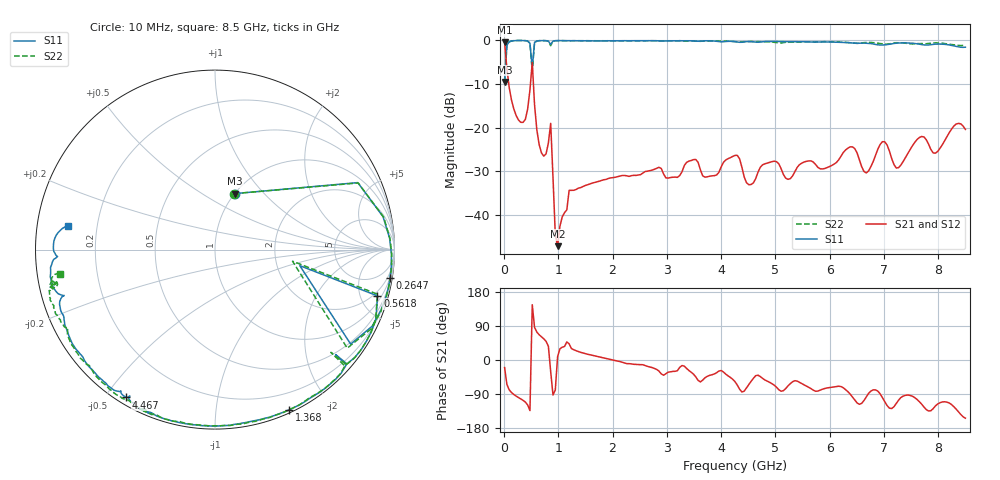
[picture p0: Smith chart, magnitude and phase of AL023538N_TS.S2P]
!AVX CORPORATION
!PN: AL023538N_TS
!DESCRIPTION: AIR CORE INDUCTOR, 538nH, 20 TURNS
!Agilent Technologies,E5071C,MY46102230,A.09.54
!Date: Mon Sep 03 16:52:48 2012
!Data & Calibration Information:
!Freq	S11:SOLT2(ON)	S21:SOLT2(ON)	S12:SOLT2(ON)	S22:SOLT2(ON)
# Hz S dB R 50
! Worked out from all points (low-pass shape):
!   201 points, 10 MHz to 8.5 GHz, reference 50 ohm
!   highest |S21| = -0.48 dB at 10 MHz (marker M1); lowest = -47.1 dB at 986.4 MHz (marker M2)
!   |S21| within 3 dB of the highest: start of sweep to 31.13 MHz
!   lowest |S11| = -9.6 dB at 10 MHz (marker M3), VSWR 1.99, Z = 50.3 + j35.3 ohm
!   |S11| at or under -10 dB: nowhere
!   |S22| runs from -9.6 to -0.1 dB; largest |S21 - S12| = 0.014
!   S11 on the Smith chart (normalised r, x): 10 MHz: 1.01, +0.71; 264.7 MHz: 1, -12; 561.9 MHz: 1.51, -6.84; 1.368 GHz: 0.03, -1.56; 4.467 GHz: 0.03, -0.57; 8.5 GHz: 0.09, +0.08
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1e7  -9.58 70.1  -0.48 -20.1  -0.61 -19.8  -9.63 71.0
5.245e7  -1.12 25.1  -6.51 -64.6  -6.48 -64.7  -1.11 25.0
2.647e8  -0.10 -9.2  -18.23 -98.9  -18.21 -99.1  -0.08 -9.6
4.7695e8  -0.71 -34.9  -11.38 -133.6  -11.37 -133.6  -0.74 -36.7
5.194e8  -6.36 -10.7  -5.09 145.9  -5.09 145.8  -7.19 -8.5
5.6185e8  -0.53 -15.9  -14.81 86.1  -14.80 86.0  -0.55 -15.4
7.3165e8  -0.12 -34.3  -26.50 55.9  -26.52 55.9  -0.12 -34.9
8.59e8  -1.00 -41.0  -19.02 -30.5  -19.02 -30.5  -1.28 -41.6
9.439e8  -0.14 -44.5  -44.41 -79.2  -44.55 -78.7  -0.15 -44.6
9.8635e8  -0.12 -47.0  -47.06 8.8  -47.34 8.4  -0.14 -47.3
1.1986e9  -0.15 -57.6  -34.32 42.7  -34.37 43.0  -0.18 -57.8
1.3684e9  -0.14 -65.1  -33.82 22.3  -33.94 22.2  -0.15 -65.4
1.4533e9  -0.16 -68.7  -33.45 18.7  -33.51 18.8  -0.15 -68.8
2.85415e9  -0.19 -110.3  -29.05 -29.3  -29.06 -29.8  -0.17 -108.3
4.255e9  -0.36 -120.1  -26.34 -57.1  -26.34 -57.3  -0.35 -135.1
4.46725e9  -0.35 -120.9  -32.57 -73.5  -32.60 -73.3  -0.35 -139.2
5.6983e9  -0.46 -140.9  -27.86 -79.6  -27.90 -80.0  -0.44 -160.8
6.41995e9  -0.66 -155.2  -24.39 -97.8  -24.40 -97.7  -0.68 -167.9
6.67465e9  -0.72 -159.7  -30.34 -97.4  -30.37 -97.2  -0.54 -167.2
7.09915e9  -0.94 -163.8  -25.30 -127.0  -25.34 -126.9  -0.85 -166.9
7.26895e9  -0.66 -167.3  -29.12 -106.0  -29.17 -105.7  -0.61 -167.7
8.5e9  -1.63 170.9  -20.40 -153.5  -20.42 -153.4  -1.19 -171.1
